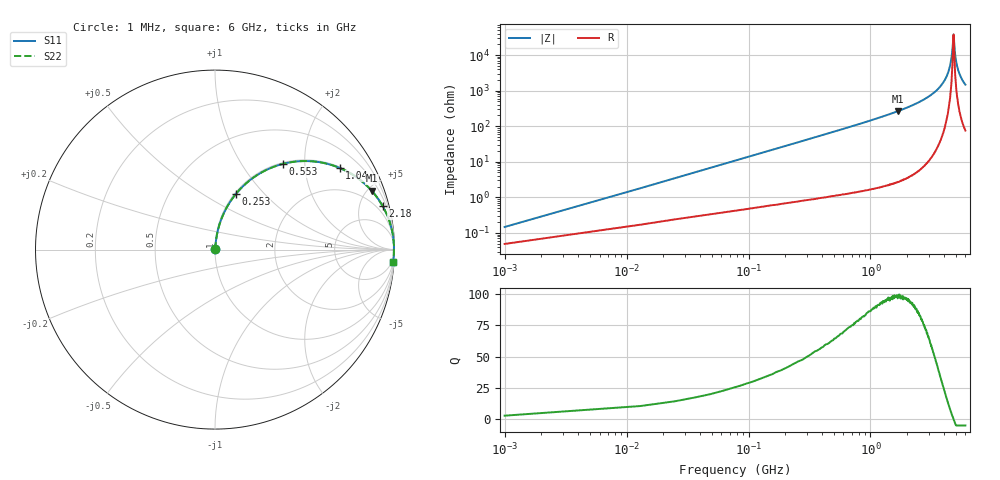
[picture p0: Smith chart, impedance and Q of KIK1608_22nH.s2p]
!version-2
!date-01.2022
!Series
# MHz S RI R 50
!Freq ReS11 ImS11 ReS21 ImS21 ReS12 ImS12 ReS22 ImS22
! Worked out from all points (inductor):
!   501 points, 1 MHz to 6 GHz, reference 50 ohm
!   read as one part in series: L = 22 nH near 25 MHz
!   highest Q = 98.2 at 1.68 GHz (marker M1), where L = 25.1 nH
!   self-resonance near 4.79 GHz
!   S11 on the Smith chart (normalised r, x): 1 MHz: 1.00, +0.00; 253 MHz: 1.02, +0.70; 553 MHz: 1.02, +1.55; 1.04 GHz: 1.03, +3.03; 2.18 GHz: 1.08, +7.62; 6 GHz: 3, -29
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1  0.000483 0.00138  0.9995 -0.00138  0.9995 -0.00138  0.000483 0.00138
37  0.00549 0.0507  0.9945 -0.0507  0.9945 -0.0507  0.00549 0.0507
61  0.0107 0.0831  0.9893 -0.0831  0.9893 -0.0831  0.0107 0.0831
133  0.0377 0.1761  0.9623 -0.1761  0.9623 -0.1761  0.0377 0.1761
253  0.1148 0.3081  0.8852 -0.3081  0.8852 -0.3081  0.1148 0.3081
553  0.3769 0.4772  0.6231 -0.4772  0.6231 -0.4772  0.3769 0.4772
1010  0.6786 0.4613  0.3214 -0.4613  0.3214 -0.4613  0.6786 0.4613
1040  0.6949 0.4548  0.3051 -0.4548  0.3051 -0.4548  0.6949 0.4548
1680  0.8727 0.3282  0.1273 -0.3282  0.1273 -0.3282  0.8727 0.3282
2020  0.9174 0.2701  0.0826 -0.2701  0.0826 -0.2701  0.9174 0.2701
2180  0.9333 0.2442  0.0667 -0.2442  0.0667 -0.2442  0.9333 0.2442
3010  0.9772 0.1418  0.0228 -0.1418  0.0228 -0.1418  0.9772 0.1418
4010  0.9948 0.0541  0.00524 -0.0541  0.00524 -0.0541  0.9948 0.0541
4350  0.9967 0.0298  0.00331 -0.0298  0.00331 -0.0298  0.9967 0.0298
4540  0.9972 0.0168  0.00278 -0.0168  0.00278 -0.0168  0.9972 0.0168
4660  0.9974 0.00901  0.00264 -0.00901  0.00264 -0.00901  0.9974 0.00901
4800  0.9974 -0.000124  0.00263 0.000124  0.00263 0.000124  0.9974 -0.000124
4940  0.9972 -0.00898  0.0028 0.00898  0.0028 0.00898  0.9972 -0.00898
5010  0.9971 -0.0126  0.00291 0.0126  0.00291 0.0126  0.9971 -0.0126
5120  0.9968 -0.0197  0.00321 0.0197  0.00321 0.0197  0.9968 -0.0197
5360  0.9959 -0.0334  0.00411 0.0334  0.00411 0.0334  0.9959 -0.0334
6000  0.992 -0.0671  0.00801 0.0671  0.00801 0.0671  0.992 -0.0671
